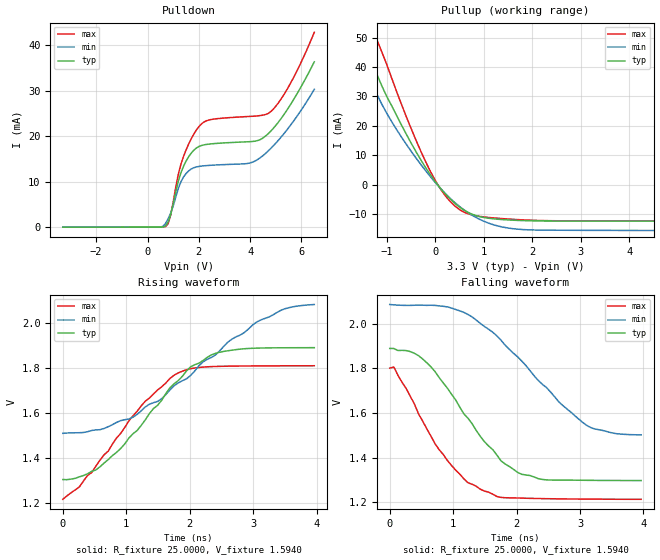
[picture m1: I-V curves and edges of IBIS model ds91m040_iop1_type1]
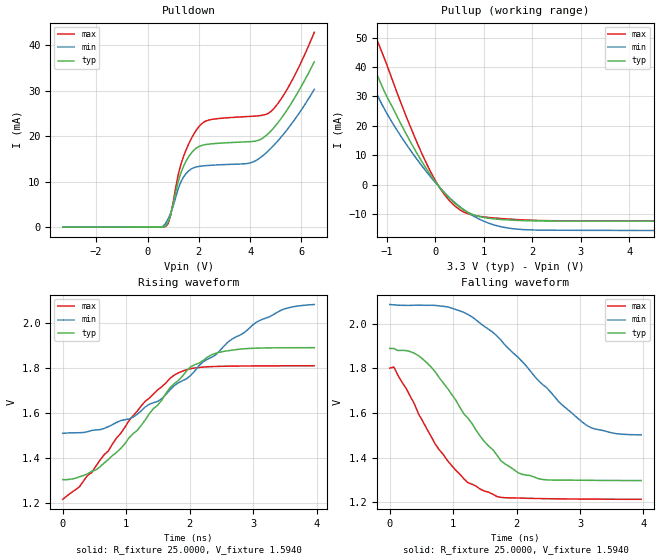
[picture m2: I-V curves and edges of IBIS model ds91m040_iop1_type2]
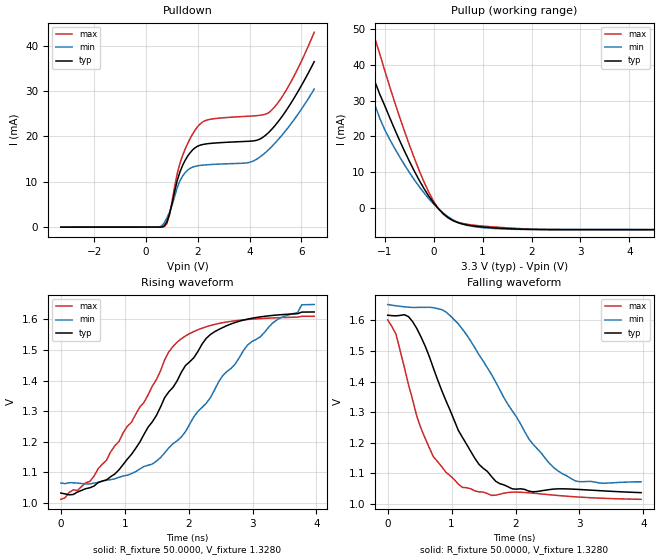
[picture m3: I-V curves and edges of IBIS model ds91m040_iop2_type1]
|   National Semiconductor Corporation
|   IBIS Model of DS91M040
[IBIS Ver]   3.2
[File name]   ds91m040.ibs
[File Rev]   1.1
[Date]   15/07/08
[Source]
[Notes]
Created by Shrikant G Kadadevar
Revision 1.1 - Updated [Pin] Construct - Shrikant K.
[Disclaimer]
(C) Copyright National Semiconductor Corporation 2008
   All rights reserved
National Semiconductor Corporation hereby grants the
user of this IBIS model a non-exclusive, nontransferable
license to use this IBIS model under the following terms.
Before using this IBIS model, the user should read this
license.  If the user does not accept these terms,  the
IBIS model should be returned to National within 30 days.
The user is granted this license only to use the
IBIS model and is not granted rights to sell, load, rent,
lease or license the IBIS model in whole or in part, or in
modified form to anyone other than user. User may modify
the IBIS model to suit its specific applications but rights
to derivative works and such modifications shall belong to
National.
This IBIS model is provided on an "AS IS" basis and
National makes absolutely no warranty with respect to the
information contained herein.NATIONAL DISCLAIMS AND CUSTOMER
WAIVES ALL WARRANTIES, EXPRESS OR IMPLIED, INCLUDING
WARRANTIES OF MERCHANTABILITY OR FITNESS FOR A PARTICULAR
PURPOSE. The entire risk as to quality and performance is
with the Customer. ACCORDINGLY, IN NO EVENT SHALL THE
COMPANY BE LIABLE FOR ANY DAMAGES, WHETHER IN CONTRACT OR
TORT,INCLUDING ANY LOST PROFITS OR OTHER INCIDENTAL,
CONSEQUENTIAL, EXEMPLARY, OR PUNITIVE DAMAGES ARISING OUT
OF THE USE OR APPLICATION OF THE IBIS model provided in
this package.Further, National reserves the right to make
changes without notice to any product herein to improve
reliability, function, or design. National does not convey
any license under patent rights or any other intellectual
property rights, including those of third parties.
National is not obligated to provide maintenance or support
for the licensed IBIS model.
[Copyright]  Copyright 2008, National Semiconductor, All Rights Reserved
[Component]  DS91M040
Si_location Pin
Timing_location Pin
[Manufacturer]  National Semiconductor Corp
[Package]
|   typ   min   max
R_pkg   0   0   0
L_pkg   0   0   0
C_pkg   0   0   0
[Pin]   signal_name   model_name   R_pin   L_pin   C_pin
1   RO1   ds91m040_cmos_out
2   DI0   ds91m040_cmos_in3
3   RO1   ds91m040_cmos_out
4   DI1   ds91m040_cmos_in3
5   RO2   ds91m040_cmos_out
6   DI2   ds91m040_cmos_in3
7   RO3   ds91m040_cmos_out
8   DI3   ds91m040_cmos_in3
9   FSEN2   ds91m040_cmos_in2
10   MDE   ds91m040_cmos_in2
11   VDD   POWER
12   VDD   POWER
13   REB1   ds91m040_cmos_in1
14   DE2   ds91m040_cmos_in1
15   REB3   ds91m040_cmos_in1
16   DE3   ds91m040_cmos_in1
17   A3   ds91m040_mlvds_iop
18   B3   ds91m040_mlvds_ion
19   A2   ds91m040_mlvds_iop
20   B2   ds91m040_mlvds_ion
21   A1   ds91m040_mlvds_iop
22   B1   ds91m040_mlvds_ion
23   A0   ds91m040_mlvds_iop
24   B0   ds91m040_mlvds_ion
25   DE0   ds91m040_cmos_in1
26   REB0   ds91m040_cmos_in1
27   DE1   ds91m040_cmos_in1
28   REB1   ds91m040_cmos_in1
29   VDD   POWER
30   VDD   POWER
31   GND   GND
32   FSEN1   ds91m040_cmos_in2
33   DAP   NC
[Diff pin]  inv_pin  vdiff  tdelay_typ  tdelay_min  tdelay_max
17 18  50m   0.0s   0.0s   0.0s
19 20  50m   0.0s   0.0s   0.0s
21 22  50m   0.0s   0.0s   0.0s
23 24  50m   0.0s   0.0s   0.0s
|Electrical package information. Will overide all the default values.
[Package Model]  LLP_32
[Model Selector]   ds91m040_mlvds_iop
ds91m040_iop1_type1   Use this model for 50-ohm loads
ds91m040_iop1_type2   Use this model for 50-ohm loads
ds91m040_iop2_type1   Use this model for 100-ohm loads
ds91m040_iop2_type2   Use this model for 100-ohm loads
[Model Selector]   ds91m040_mlvds_ion
ds91m040_ion1_type1   Use this model for 50-ohm loads
ds91m040_ion1_type2   Use this model for 50-ohm loads
ds91m040_ion2_type1   Use this model for 100-ohm loads
ds91m040_ion2_type2   Use this model for 100-ohm loads
| Elecrical Package Models
[Define Package Model]  LLP_32
[Manufacturer]   National Semiconductor
[OEM]   NA
[Description]   32 LLP for DS91M040 at 125MHz frequency
[Number Of Pins]   33
[Pin Numbers]
   1   |   1 = L1
   2   |   2 = L2
   3   |   3 = L3
   4   |   4 = L4
   5   |   5 = L5
   6   |   6 = L6
   7   |   7 = L7
   8   |   8 = L8
   9   |   9 = L9
  10   |  10 = L10
  11   |  11 = L11
  12   |  12 = L12
  13   |  13 = L13
  14   |  14 = L14
  15   |  15 = L15
  16   |  16 = L16
  17   |  17 = L17
  18   |  18 = L18
  19   |  19 = L19
  20   |  20 = L20
  21   |  21 = L21
  22   |  22 = L22
  23   |  23 = L23
  24   |  24 = L24
  25   |  25 = L25
  26   |  26 = L26
  27   |  27 = L27
  28   |  28 = L28
  29   |  29 = L29
  30   |  30 = L30
  31   |  31 = L31
  32   |  32 = L32
  33   |  33 = L_DAP
[Model Data]
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[End Model Data]
[End Package Model]
| Models and submodels in the file (12): ds91m040_iop1_type1 (I/O), ds91m040_iop1_type2 (I/O), ds91m040_iop2_type1 (I/O), ds91m040_iop2_type2 (I/O), ds91m040_ion1_type1 (I/O), ds91m040_ion1_type2 (I/O), ds91m040_ion2_type1 (I/O), ds91m040_ion2_type2 (I/O), ds91m040_cmos_out (Output), ds91m040_cmos_in1 (Input), ds91m040_cmos_in2 (Input), ds91m040_cmos_in3 (Input)
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|   Model ds91m040_iop1_type1
[Model]  ds91m040_iop1_type1
Model_type I/O
Polarity   Non-Inverting
Vinl = -0.05
Vinh = +0.05
Vmeas =  1.56V
Rref =   25.0000
Vref =   1.56V
C_comp   7.359p   6.991p  7.743p
[Model Spec]
S_overshoot_high   3.8   3.8   3.8
S_overshoot_low   -1.4   -1.4   -1.4
[Temperature Range]   25.0000   85.0000   -40.0000
[Voltage Range]   3.3000V   3.0000V   3.6000V
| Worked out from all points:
|   slope of the pullup table from 0 to 0.495 V, typ, clamps not added: 57.8 ohm
|   rising waveform, R_fixture 25.0000, V_fixture 1.5940: 20-80 % time 1.08ns typ, 1.61ns min, 1ns max; typ from 1.3 V to 1.89 V
|   falling waveform, R_fixture 25.0000, V_fixture 1.5940: 20-80 % time 928ps typ, 1.2ns min, 780ps max; typ from 1.89 V to 1.3 V
[Pulldown]
|Voltage   I(typ)   I(min)   I(max)
-3.3V     -16.04uA   -15.04uA   -17.07uA
500mV     -2.06uA    10.82uA    -4.562uA
700mV     234.6uA    784.7uA    91.14uA
900mV     2.713mA    3.039mA    2.586mA
1.2V      10.09mA    8.499mA    11.63mA
1.4V      13.34mA    10.98mA    15.49mA
2V        17.72mA    13.33mA    22.08mA
2.5V      18.31mA    13.61mA    23.68mA
4V        18.79mA    14.11mA    24.35mA
4.8V      21.08mA    17.27mA    25.39mA
5.6V      27.19mA    22.62mA    31.92mA
6.5V      36.35mA    30.31mA    42.84mA
[Pullup]
|Voltage   I(typ)   I(min)   I(max)
-3.3V     175.7mA    142.4mA    190.6mA
-1.7V     63.82mA    53.26mA    77.6mA
-1.5V     51.44mA    43.29mA    64.96mA
-1.3V     41.45mA    34.36mA    54.06mA
-800mV    23.56mA    18.75mA    31.69mA
-400mV    11.23mA    9.085mA    15.15mA
-100mV    3.299mA    2.667mA    4.432mA
200mV     -3.058mA   -2.926mA   -3.666mA
600mV     -8.75mA    -8.684mA   -9.419mA
1.2V      -11.61mA   -13.63mA   -11.3mA
1.8V      -12.2mA    -15.25mA   -11.96mA
6.5V      -12.39mA   -15.63mA   -12.32mA
[Ramp]
| variable   typ   min   max
dV/dt_r  0.3567/1.100n   0.3514/1.640n   0.3599/1.010n
dV/dt_f  0.3578/0.936n   0.3457/1.180n   0.3610/0.798n
R_load = 25.00
[Rising Waveform]
R_fixture= 25.0000
V_fixture= 1.5940
V_fixture_min= 1.7950
V_fixture_max= 1.5120
|time   V(typ)   V(min)   V(max)
0s        1.303V     1.509V     1.215V
260ps     1.315V     1.512V     1.27V
585ps     1.36V      1.526V     1.389V
1.3ns     1.569V     1.627V     1.652V
1.82ns    1.745V     1.734V     1.779V
2.015ns   1.806V     1.768V     1.798V
2.47ns    1.871V     1.876V     1.808V
3.12ns    1.89V      2.015V     1.81V
3.51ns    1.891V     2.066V     1.81V
3.965ns   1.891V     2.084V     1.811V
[Falling Waveform]
R_fixture= 25.0000
V_fixture= 1.5940
V_fixture_min= 1.7950
V_fixture_max= 1.5120
|time   V(typ)   V(min)   V(max)
0s        1.889V     2.086V     1.801V
65ps      1.889V     2.084V     1.806V
585ps     1.825V     2.082V     1.529V
975ps     1.684V     2.07V      1.365V
1.43ns    1.495V     2.001V     1.259V
1.755ns   1.386V     1.926V     1.223V
2.08ns    1.326V     1.833V     1.219V
2.665ns   1.3V       1.651V     1.216V
3.12ns    1.299V     1.542V     1.215V
3.965ns   1.298V     1.502V     1.214V
|   Model ds91m040_iop1_type2
[Model]  ds91m040_iop1_type2
Model_type I/O
Polarity   Non-Inverting
Vinl = 0.05
Vinh = 0.15
Vmeas =  1.56V
Rref =   25.0000
Vref =   1.56V
C_comp   7.359p   6.991p  7.743p
[Model Spec]
S_overshoot_high   3.8   3.8   3.8
S_overshoot_low   -1.4   -1.4   -1.4
[Temperature Range]   25.0000   85.0000   -40.0000
[Voltage Range]   3.3000V   3.0000V   3.6000V
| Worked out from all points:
|   slope of the pullup table from 0 to 0.495 V, typ, clamps not added: 57.8 ohm
|   rising waveform, R_fixture 25.0000, V_fixture 1.5940: 20-80 % time 1.08ns typ, 1.61ns min, 1ns max; typ from 1.3 V to 1.89 V
|   falling waveform, R_fixture 25.0000, V_fixture 1.5940: 20-80 % time 928ps typ, 1.2ns min, 780ps max; typ from 1.89 V to 1.3 V
[Pulldown]
|Voltage   I(typ)   I(min)   I(max)
-3.3V     -16.04uA   -15.04uA   -17.07uA
500mV     -2.06uA    10.82uA    -4.562uA
700mV     234.6uA    784.7uA    91.14uA
900mV     2.713mA    3.039mA    2.586mA
1.2V      10.09mA    8.499mA    11.63mA
1.4V      13.34mA    10.98mA    15.49mA
2V        17.72mA    13.33mA    22.08mA
2.5V      18.31mA    13.61mA    23.68mA
4V        18.79mA    14.11mA    24.35mA
4.8V      21.08mA    17.27mA    25.39mA
5.6V      27.19mA    22.62mA    31.92mA
6.5V      36.35mA    30.31mA    42.84mA
[Pullup]
|Voltage   I(typ)   I(min)   I(max)
-3.3V     175.7mA    142.4mA    190.6mA
-1.7V     63.82mA    53.26mA    77.6mA
-1.5V     51.44mA    43.29mA    64.96mA
-1.3V     41.45mA    34.36mA    54.06mA
-800mV    23.56mA    18.75mA    31.69mA
-400mV    11.23mA    9.085mA    15.15mA
-100mV    3.299mA    2.667mA    4.432mA
200mV     -3.058mA   -2.926mA   -3.666mA
600mV     -8.75mA    -8.684mA   -9.419mA
1.2V      -11.61mA   -13.63mA   -11.3mA
1.8V      -12.2mA    -15.25mA   -11.96mA
6.5V      -12.39mA   -15.63mA   -12.32mA
[Ramp]
| variable   typ   min   max
dV/dt_r  0.3567/1.100n   0.3514/1.640n   0.3599/1.010n
dV/dt_f  0.3578/0.936n   0.3457/1.180n   0.3610/0.798n
R_load = 25.00
[Rising Waveform]
R_fixture= 25.0000
V_fixture= 1.5940
V_fixture_min= 1.7950
V_fixture_max= 1.5120
|time   V(typ)   V(min)   V(max)
0s        1.302V     1.509V     1.215V
260ps     1.315V     1.512V     1.27V
585ps     1.36V      1.526V     1.389V
1.3ns     1.569V     1.627V     1.652V
1.82ns    1.745V     1.734V     1.779V
2.015ns   1.806V     1.768V     1.798V
2.47ns    1.871V     1.876V     1.808V
3.12ns    1.89V      2.015V     1.81V
3.51ns    1.891V     2.066V     1.81V
3.965ns   1.891V     2.084V     1.811V
[Falling Waveform]
R_fixture= 25.0000
V_fixture= 1.5940
V_fixture_min= 1.7950
V_fixture_max= 1.5120
|time   V(typ)   V(min)   V(max)
0s        1.889V     2.086V     1.801V
65ps      1.889V     2.084V     1.806V
585ps     1.825V     2.082V     1.529V
975ps     1.684V     2.07V      1.365V
1.43ns    1.495V     2.001V     1.259V
1.755ns   1.386V     1.926V     1.223V
2.08ns    1.326V     1.833V     1.219V
2.665ns   1.3V       1.651V     1.216V
3.12ns    1.299V     1.542V     1.215V
3.965ns   1.298V     1.502V     1.214V
|   Model ds91m040_iop2_type1
[Model] ds91m040_iop2_type1
Model_type I/O
Polarity   Non-Inverting
Vinl = -0.05
Vinh = 0.05
Vmeas =  1.56V
Rref =   50.0000
Vref =   1.56V
C_comp   7.359p   6.991p  7.743p
[Model Spec]
S_overshoot_high   3.8   3.8   3.8
S_overshoot_low   -1.4   -1.4   -1.4
[Temperature Range]   25.0000   85.0000   -40.0000
[Voltage Range]   3.3000V   3.0000V   3.6000V
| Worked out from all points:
|   slope of the pullup table from 0 to 0.495 V, typ, clamps not added: 89.8 ohm
|   rising waveform, R_fixture 50.0000, V_fixture 1.3280: 20-80 % time 1.1ns typ, 1.33ns min, 1.01ns max; typ from 1.03 V to 1.62 V
|   falling waveform, R_fixture 50.0000, V_fixture 1.3280: 20-80 % time 738ps typ, 1.02ns min, 589ps max; typ from 1.62 V to 1.04 V
[Pulldown]
|Voltage   I(typ)   I(min)   I(max)
-3.3V     -16.03uA   -15.03uA   -17.07uA
500mV     -1.779uA   19.11uA    -4.505uA
700mV     266.1uA    947.9uA    95.95uA
900mV     2.789mA    3.225mA    2.636mA
1.2V      10.22mA    8.651mA    11.74mA
1.4V      13.49mA    11.17mA    15.63mA
2V        17.87mA    13.53mA    22.22mA
2.5V      18.47mA    13.8mA     23.81mA
4V        18.95mA    14.28mA    24.48mA
4.8V      21.23mA    17.43mA    25.52mA
5.6V      27.34mA    22.77mA    32.05mA
6.5V      36.5mA     30.45mA    42.97mA
[Pullup]
|Voltage   I(typ)   I(min)   I(max)
-3.3V     175.6mA    142.3mA    190.5mA
-1.7V     63.38mA    52.81mA    76.23mA
-1.6V     56.8mA     47.64mA    68.59mA
-1.5V     50.5mA     42.58mA    62.09mA
-1.3V     39.51mA    33.04mA    51.53mA
-1.2V     35.24mA    28.74mA    47.34mA
-900mV    25.28mA    19.17mA    33.99mA
-200mV    5.404mA    4.186mA    7.28mA
100mV     -330.9uA   -343uA     -296.8uA
500mV     -4.222mA   -4.121mA   -4.112mA
1.6V      -5.915mA   -6.038mA   -5.727mA
6.5V      -6.152mA   -6.146mA   -6.187mA
[Ramp]
| variable   typ   min   max
dV/dt_r  0.3571/1.190n   0.3519/1.440n   0.3593/1.070n
dV/dt_f  0.3557/0.812n   0.3514/1.110n   0.3588/0.645n
R_load = 50.00
[Rising Waveform]
R_fixture= 50.0000
V_fixture= 1.3280
V_fixture_min= 1.3569
V_fixture_max= 1.3117
|time   V(typ)   V(min)   V(max)
0s        1.032V     1.065V     1.011V
455ps     1.049V     1.062V     1.07V
845ps     1.094V     1.078V     1.186V
1.43ns    1.264V     1.127V     1.381V
1.69ns    1.363V     1.18V      1.494V
1.885ns   1.427V     1.215V     1.537V
2.275ns   1.538V     1.325V     1.576V
2.6ns     1.58V      1.43V      1.592V
3.315ns   1.613V     1.589V     1.605V
3.965ns   1.625V     1.649V     1.61V
[Falling Waveform]
R_fixture= 50.0000
V_fixture= 1.3280
V_fixture_min= 1.3569
V_fixture_max= 1.3117
|time   V(typ)   V(min)   V(max)
0s        1.617V     1.652V     1.601V
130ps     1.615V     1.647V     1.554V
325ps     1.612V     1.643V     1.39V
650ps     1.482V     1.643V     1.184V
1.17ns    1.218V     1.571V     1.054V
1.755ns   1.066V     1.373V     1.032V
2.21ns    1.042V     1.212V     1.037V
2.6ns     1.049V     1.119V     1.029V
2.99ns    1.047V     1.073V     1.023V
3.965ns   1.037V     1.072V     1.015V
